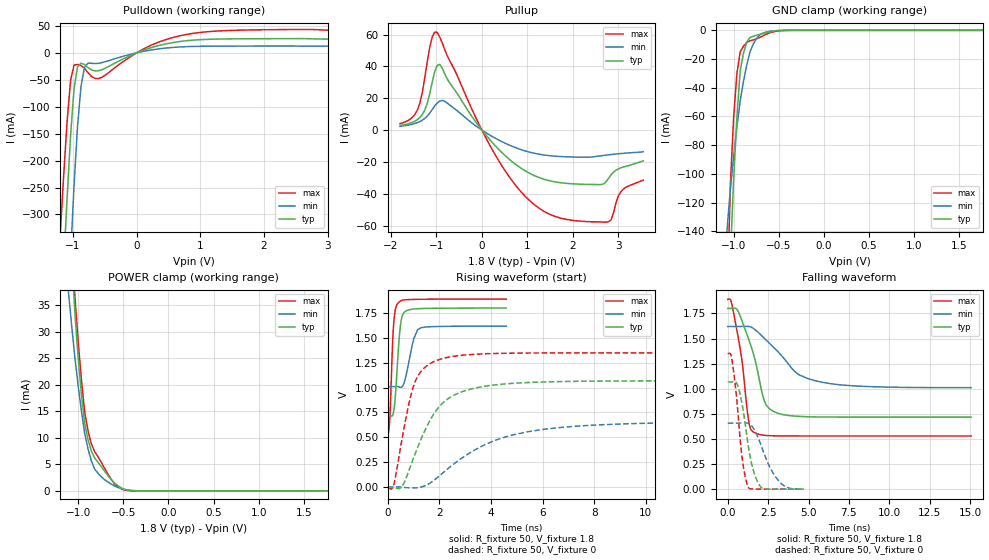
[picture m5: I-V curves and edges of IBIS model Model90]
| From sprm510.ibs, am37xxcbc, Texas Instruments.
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| Model based on original model for BQ18OMAPSMART1HYFBPBNOPM_SSBHV
|   Sub model PM_VS01L01_PUPD0_1P8
[model]   Model90
|[Input Load]   PI
|[Output Drive] SC01LB01
|Voltage   1.8V
|Mode   I/O
Model_type   I/O
Polarity   Non-Inverting
Enable   Active-Low
Vinl =  0.63
Vinh =  1.17
Cref =  15pF
Rref =  100.0000M
Vref =  0V
Vmeas =  0.9
C_comp   1.410688p   1.256095p   1.577871p
[Model Spec]
Vinl   0.63   0.567   0.6615
Vinh   1.17   1.053   1.2285
[Temperature Range]   25   125   -40
[Voltage Range]   1.8   1.62   1.89
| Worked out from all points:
|   slope of the pulldown table from 0 to 0.27 V, typ, clamps not added: 24.3 ohm
|   slope of the pullup table from 0 to 0.27 V, typ, clamps not added: 29.7 ohm
|   GND clamp passes 1 mA (typ) near -0.60 V on its own axis
|   POWER clamp passes 1 mA (typ) near -0.56 V on its own axis
|   rising waveform, R_fixture 50, V_fixture 1.8: 20-80 % time 175ps typ, 302ps min, 124ps max; typ from 0.717 V to 1.8 V
|   rising waveform, R_fixture 50, V_fixture 0: 20-80 % time 1.29ns typ, 2.78ns min, 687ps max; typ from 0 V to 1.07 V
|   falling waveform, R_fixture 50, V_fixture 1.8: 20-80 % time 1.07ns typ, 2.2ns min, 671ps max; typ from 1.8 V to 0.718 V
|   falling waveform, R_fixture 50, V_fixture 0: 20-80 % time 662ps typ, 1.07ns min, 491ps max; typ from 1.07 V to 0 V
[POWER_clamp]
-1.8V     362.5mA    191.4mA    412.8mA
-1.109V   56.69mA    37.71mA    60.38mA
-1.073V   44.6mA     31.22mA    47.8mA
-1.036V   33.44mA    25.04mA    36.59mA
-1V       24.98mA    19.72mA    28.06mA
-963.6mV  18.03mA    14.96mA    20.78mA
-927.3mV  12.59mA    10.77mA    14.74mA
-890.9mV  9.653mA    7.899mA    11.31mA
-818.2mV  6.214mA    4.114mA    7.414mA
-636.4mV  2.183mA    1.307mA    2.238mA
-418.2mV  83.85uA    105.2uA    35.14uA
1.764V    -1.228nA   -79.11nA   -1.453nA
[Pulldown]
-1.8V     -1.718A    -2.61A     -1.406A
-1.2V     -527.4mA   -844.5mA   -339.9mA
-1.145V   -396mA     -683.1mA   -229.1mA
-1.091V   -269mA     -526.7mA   -127.5mA
-1.036V   -153.6mA   -378.9mA   -51.17mA
-981.8mV  -66.34mA   -245.6mA   -22.67mA
-927.3mV  -26mA      -136.2mA   -21.54mA
-872.7mV  -19.34mA   -61.98mA   -23.69mA
-763.6mV  -27.2mA    -19.05mA   -36.72mA
-545.5mV  -31.39mA   -18.17mA   -45.46mA
872.7mV   23.46mA    11.88mA    35.92mA
3.545V    25.34mA    12.51mA    41.58mA
[Pullup]
-1.8V     2.903mA    2.423mA    4.112mA
-1.418V   6.595mA    4.711mA    12.64mA
-1.255V   12.69mA    7.42mA     33.23mA
-1.091V   30.4mA     13mA       58.69mA
-981.8mV  40.63mA    17.02mA    61.3mA
-818.2mV  35.38mA    18.12mA    50.59mA
272.7mV   -9.18mA    -4.728mA   -14.55mA
1.255V    -29.75mA   -15.09mA   -48.97mA
2.564V    -34.17mA   -16.31mA   -57.57mA
2.782V    -30.25mA   -15.5mA    -57.48mA
3.055V    -23.63mA   -14.68mA   -38.61mA
3.545V    -19.25mA   -13.56mA   -31.41mA
[GND_clamp]
-1.8V     -2.82A     -1.192A    -3.165A
-1.073V   -235.7mA   -138.4mA   -192.1mA
-1.036V   -159.5mA   -110.8mA   -107.5mA
-1V       -103.8mA   -87.85mA   -60.67mA
-963.6mV  -60mA      -67.28mA   -29.8mA
-927.3mV  -28.21mA   -49.08mA   -14.9mA
-890.9mV  -15.9mA    -35.48mA   -10.99mA
-854.5mV  -8.138mA   -24.07mA   -8.449mA
-818.2mV  -4.924mA   -14.85mA   -7.266mA
-709.1mV  -2.784mA   -3.064mA   -4.883mA
-563.6mV  -570.2uA   -404.5uA   -1.092mA
1.764V    -11.02pA   583.5nA    3.035nA
[Ramp]
dV/dt_f  0.6512583/1.074538n   0.3676939/2.220695n   0.8182458/0.6731533n
dV/dt_r  0.6509731/1.288404n   0.4007486/2.803131n   0.8227645/0.6885725n
R_load = 50
[Rising Waveform]
R_fixture = 50
V_fixture = 1.8
V_fixture_min = 1.62
V_fixture_max = 1.89
0s        717.3mV    1.009V     527.8mV
81ps      719.4mV    1.009V     720.1mV
180ps     718.7mV    1.009V     1.428V
234ps     774mV      1.009V     1.672V
396ps     1.34V      1.01V      1.851V
486ps     1.624V     1.002V     1.87V
567ps     1.726V     1.013V     1.878V
999ps     1.79V      1.486V     1.886V
1.152ns   1.793V     1.582V     1.887V
4.59ns    1.799V     1.618V     1.89V
[Rising Waveform]
R_fixture = 50
V_fixture = 0
V_fixture_min = 0
V_fixture_max = 0
0s        158.4uV    102uV      -10.85mV
225ps     -9.968mV   -202.3uV   17.7mV
585ps     19.94mV    -4.018mV   535mV
855ps     193mV      -8.514mV   881.3mV
1.08ns    349.7mV    -10.05mV   1.072V
1.611ns   659.2mV    34.83mV    1.236V
2.097ns   836.9mV    133.8mV    1.29V
3.915ns   1.019V     442.6mV    1.341V
6.057ns   1.056V     580mV      1.348V
19.18ns   1.067V     655.8mV    1.349V
[Falling Waveform]
R_fixture = 50
V_fixture = 1.8
V_fixture_min = 1.62
V_fixture_max = 1.89
0s        1.8V       1.62V      1.89V
297ps     1.802V     1.62V      1.81V
837ps     1.695V     1.621V     1.328V
1.323ns   1.48V      1.62V      654mV
1.62ns    1.329V     1.598V     566.4mV
2.268ns   877.6mV    1.502V     536.6mV
3.204ns   751.4mV    1.353V     530.6mV
4.374ns   725.5mV    1.144V     529.8mV
5.814ns   718.9mV    1.065V     529.8mV
15.06ns   717.6mV    1.011V     529.8mV
[Falling Waveform]
R_fixture = 50
V_fixture = 0
V_fixture_min = 0
V_fixture_max = 0
0s        1.068V     657.2mV    1.349V
270ps     1.07V      657.5mV    1.279V
648ps     1.017V     657.8mV    725.9mV
945ps     793mV      661.1mV    246.6mV
1.287ns   412.5mV    654.5mV    15.61mV
1.602ns   178.4mV    603.2mV    1.833mV
2.079ns   16.15mV    430.1mV    231.7uV
2.628ns   1.568mV    211.9mV    27.03uV
3.285ns   340.4uV    60.32mV    3.518uV
4.707ns   51.92uV    1.646mV    458nV
